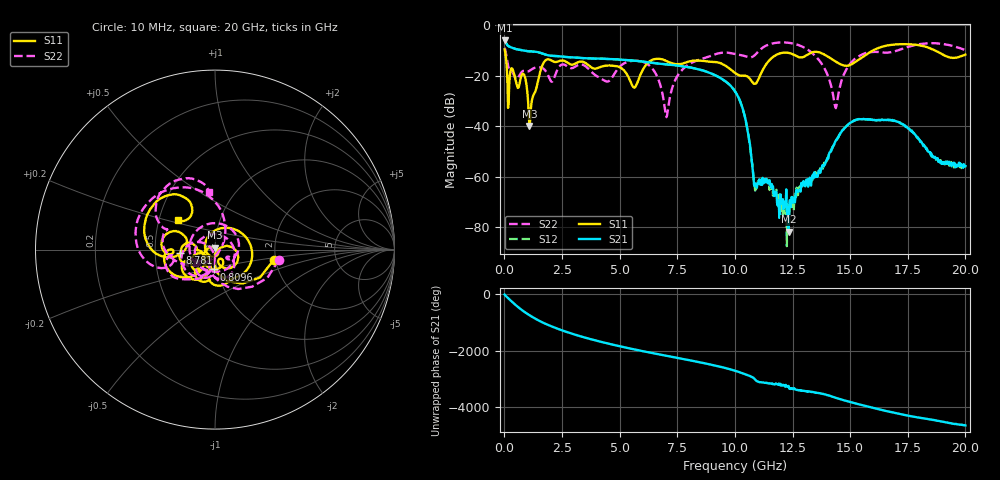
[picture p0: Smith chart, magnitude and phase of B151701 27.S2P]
!  2-Port S-parameters saved by WinCal
! VAR MeasName=S-Parameters (CALIBRATED_DATA) read from VNA (N5244A)
! VAR MeasDate=2015-12-24 19:11:16
! VAR NAME=B151701 27
! VAR FILENAME=B151701 27.S2P
! VAR DATE=2015-12-24 19:11:16
! VAR PHYS_PORTS=1,3
# Hz S DB R 50
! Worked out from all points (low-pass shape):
!   801 points, 10 MHz to 20 GHz, reference 50 ohm
!   highest |S21| = -5.97 dB at 10 MHz (marker M1); lowest = -81.8 dB at 12.33 GHz (marker M2)
!   |S21| within 3 dB of the highest: start of sweep to 371.2 MHz
!   lowest |S11| = -39.9 dB at 1.084 GHz (marker M3), VSWR 1.02, Z = 50.1 + j1.01 ohm
!   |S11| at or under -10 dB: 20.59 MHz to 15.98 GHz (15.96 GHz wide, 199 % of centre); 18.7 GHz to end of sweep
!   |S22| runs from -36.3 to -6.7 dB; largest |S21 - S12| = 0.0011
!   S11 on the Smith chart (normalised r, x): 10 MHz: 1.96, -0.25; 809.6 MHz: 0.96, -0.21; 8.781 GHz: 0.68, -0.02; 20 GHz: 0.63, +0.22
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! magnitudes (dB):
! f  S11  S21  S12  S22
! 10 MHz  -9.6  -6.0  -6.0  -8.9
! 209.9 MHz  -23.3  -8.4  -8.4  -17.5
! 809.6 MHz  -19.1  -9.9  -9.9  -18.1
! 1.084 GHz  -39.9  -10.3  -10.3  -18.0
! 1.784 GHz  -13.8  -11.6  -11.6  -18.0
! 3.358 GHz  -14.3  -12.9  -12.9  -15.5
! 4.458 GHz  -15.9  -13.3  -13.3  -22.2
! 5.632 GHz  -24.7  -14.0  -14.0  -14.0
! 6.682 GHz  -13.2  -15.1  -15.1  -21.4
! 7.031 GHz  -14.1  -15.4  -15.4  -36.3
! 7.606 GHz  -15.3  -16.0  -16.0  -18.8
! 8.781 GHz  -14.2  -18.4  -18.4  -12.6
! 10.01 GHz  -18.8  -26.1  -26.1  -11.3
! 10.43 GHz  -19.9  -36.0  -36.1  -12.1
! 10.9 GHz  -23.1  -62.8  -62.8  -11.4
! 11.38 GHz  -15.1  -61.2  -60.9  -7.9
! 12.33 GHz  -10.9  -81.8  -72.0  -6.9
! 13.35 GHz  -10.7  -60.4  -59.9  -11.0
! 14.38 GHz  -14.3  -45.7  -45.8  -32.8
! 15.13 GHz  -15.1  -37.9  -38.0  -13.9
! 16.68 GHz  -7.8  -37.6  -37.4  -10.7
! 20 GHz  -11.6  -55.7  -56.4  -9.8
